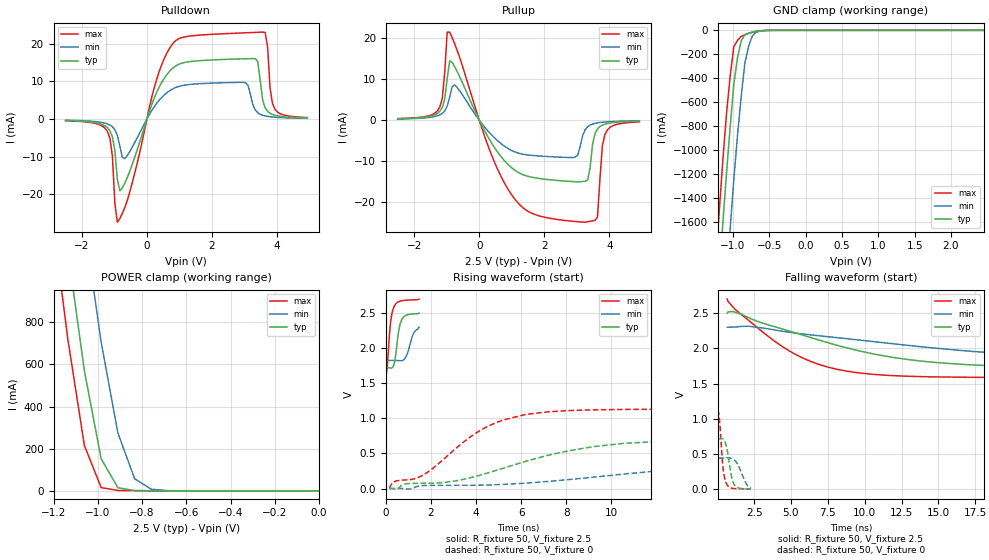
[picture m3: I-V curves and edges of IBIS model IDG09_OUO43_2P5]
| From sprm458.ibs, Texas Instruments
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|IDG09_OUO43_2P75; DEFAULT
|   Model Cell IDG09_OUO43_2P5
|IDG09_OUO43_2P5
[Model]   IDG09_OUO43_2P5
Model_type   I/O
Polarity   Non-Inverting
Enable   Active-Low
Vinl =  0.7V
Vinh =  1.7V
Cref =  15pF
Rref =  100.00M
Vref =  0V
Vmeas =  1.25
C_comp   3.099p   3.082p   3.128p
[Model Spec]
Vinl   0.7V   0.7V   0.7V
Vinh   1.7V   1.7V   1.7V
[Temperature Range]   25   125   -40
[Voltage Range]   2.5   2.3   2.7
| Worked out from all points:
|   slope of the pulldown table from 0 to 0.375 V, typ, clamps not added: 44.4 ohm
|   slope of the pullup table from 0 to 0.375 V, typ, clamps not added: 67.8 ohm
|   GND clamp passes 1 mA (typ) near -0.54 V on its own axis
|   POWER clamp passes 1 mA (typ) near -0.78 V on its own axis
|   rising waveform, R_fixture 50, V_fixture 2.5: 20-80 % time 209ps typ, 269ps min, 183ps max; typ from 1.72 V to 2.5 V
|   rising waveform, R_fixture 50, V_fixture 0: 20-80 % time 5.09ns typ, 9.64ns min, 2.82ns max; typ from 0 V to 0.711 V
|   falling waveform, R_fixture 50, V_fixture 2.5: 20-80 % time 8.46ns typ, 14ns min, 4.75ns max; typ from 2.5 V to 1.72 V
|   falling waveform, R_fixture 50, V_fixture 0: 20-80 % time 346ps typ, 555ps min, 257ps max; typ from 0.711 V to 0 V
[POWER_clamp]
|   voltage   I(typ)   I(min)   I(max)
-2.5V     14.14A     14.81A     13.77A
-1.162V   1.362A     2.103A     937.6mA
-1.111V   954.8mA    1.678A     556.6mA
-1.061V   569.9mA    1.264A     215.7mA
-1.035V   430.8mA    1.078A     149.1mA
-1.01V    291.8mA    892.4mA    82.46mA
-984.8mV  152.7mA    706.5mA    15.84mA
-909.1mV  14.92mA    274.3mA    2.264mA
-833.3mV  1.74mA     57.42mA    1.347mA
-757.6mV  686.5uA    7.849mA    844.3uA
-681.8mV  369.5uA    1.246mA    453.6uA
0V        47.1pA     7.855nA    439.6fA
[Pulldown]
|   voltage   I(typ)   I(min)   I(max)
-2.5V     -389.7uA   -297.8uA   -436.3uA
-1.212V   -2.281mA   -1.295mA   -3.317mA
-1.061V   -4.693mA   -2.054mA   -9.806mA
-909.1mV  -15.92mA   -4.294mA   -27.38mA
-681.8mV  -17.04mA   -10.53mA   -23.54mA
303mV     7.158mA    4.194mA    10.64mA
984.8mV   14.58mA    8.68mA     21.35mA
3.03V     16.01mA    9.688mA    22.91mA
3.333V    16.04mA    2.419mA    23.01mA
3.636V    2.972mA    843.8uA    23mA
3.939V    1.009mA    493.8uA    2.614mA
4.924V    304.5uA    206.1uA    415.7uA
[Pullup]
|   voltage   I(typ)   I(min)   I(max)
-2.5V     313.5uA    255.7uA    361.5uA
-1.212V   2.129mA    1.281mA    3.17mA
-984.8mV  10.18mA    3.39mA     21.48mA
-909.1mV  14.47mA    5.593mA    21.51mA
-757.6mV  13.07mA    8.592mA    18.68mA
984.8mV   -11.57mA   -7.382mA   -18.14mA
2.955V    -15.07mA   -9.072mA   -24.8mA
3.258V    -14.97mA   -2.349mA   -24.97mA
3.636V    -2.169mA   -686.5uA   -23.72mA
3.788V    -1.243mA   -526uA     -6.264mA
3.939V    -859.3uA   -425.2uA   -2.43mA
4.924V    -278.6uA   -187uA     -439.4uA
[GND_clamp]
|   voltage   I(typ)   I(min)   I(max)
-2.5V     -14.67A    -15.53A    -14.19A
-1.237V   -2.509A    -3.422A    -1.974A
-1.187V   -2.057A    -2.967A    -1.526A
-1.136V   -1.613A    -2.517A    -1.089A
-1.035V   -807.8mA   -1.658A    -382.1mA
-984.8mV  -448.6mA   -1.246A    -135.7mA
-934.3mV  -228.2mA   -878.6mA   -83.75mA
-883.8mV  -90.46mA   -554.2mA   -50.81mA
-833.3mV  -35.41mA   -273.2mA   -36.84mA
-782.8mV  -24.03mA   -135.4mA   -25.97mA
-681.8mV  -8.733mA   -15.88mA   -8.435mA
2.449V    45.65pA    49.92nA    439.6fA
[Ramp]
| variable   typ   min   max
dV/dt_f 0.48022702/8.6079833n 0.29244605/14.147187n  0.6869356/4.8204991n
dV/dt_r 0.43192829/5.1069038n 0.26821048/9.6318823n 0.68422665/2.8447429n
R_load = 50
[Rising Waveform]
R_fixture = 50
V_fixture = 2.5
V_fixture_min = 2.3
V_fixture_max = 2.7
|   time   V(typ)   V(min)   V(max)
0s        1.722V     1.826V     1.586V
69.15ps   1.722V     1.826V     1.769V
204.2ps   1.718V     1.826V     2.352V
346.8ps   1.756V     1.826V     2.579V
421.7ps   1.869V     1.825V     2.624V
578.6ps   2.264V     1.823V     2.664V
708.6ps   2.408V     1.822V     2.676V
914.8ps   2.471V     1.892V     2.684V
1.222ns   2.488V     2.206V     2.689V
1.473ns   2.5V       2.3V       2.7V
[Rising Waveform]
R_fixture = 50
V_fixture = 0
V_fixture_min = 0
V_fixture_max = 0
|   time   V(typ)   V(min)   V(max)
169.3ps   55.05pV    16.04nV    1.076pV
409.9ps   -8.199mV   226.2uV    101.9mV
863.9ps   64.11mV    -3.231mV   121.9mV
1.811ns   74.84mV    44.11mV    223.7mV
4.401ns   210.1mV    49.62mV    866.3mV
6.166ns   383.7mV    75.74mV    1.053V
8.051ns   533.7mV    125.2mV    1.11V
10.6ns    645.2mV    207.2mV    1.127V
14.55ns   698.1mV    319.8mV    1.13V
22.97ns   710.6mV    439.6mV    1.13V
[Falling Waveform]
R_fixture = 50
V_fixture = 2.5
V_fixture_min = 2.3
V_fixture_max = 2.7
|   time   V(typ)   V(min)   V(max)
678.7ps   2.5V       2.3V       2.7V
1.374ns   2.502V     2.306V     2.525V
2.23ns    2.426V     2.312V     2.379V
4.484ns   2.271V     2.241V     2.016V
6.335ns   2.154V     2.192V     1.814V
8.156ns   2.042V     2.151V     1.701V
11.87ns   1.873V     2.067V     1.613V
14.87ns   1.798V     2.001V     1.594V
25.31ns   1.728V     1.869V     1.587V
25.68ns   1.722V     1.826V     1.586V
[Falling Waveform]
R_fixture = 50
V_fixture = 0
V_fixture_min = 0
V_fixture_max = 0
|   time   V(typ)   V(min)   V(max)
63.27ps   710.6mV    439.6mV    1.13V
164.6ps   717.1mV    439.6mV    953.3mV
386.1ps   713.9mV    442.9mV    313.6mV
481.8ps   690.9mV    444.6mV    176.1mV
593.6ps   631.4mV    446.3mV    93.55mV
966.3ps   181.4mV    436.6mV    15.43mV
1.132ns   71.92mV    416.4mV    9.41mV
1.444ns   17.59mV    329.8mV    5.187mV
1.929ns   4.903mV    93.12mV    2.707mV
2.26ns    55.05pV    16.04nV    1.076pV
